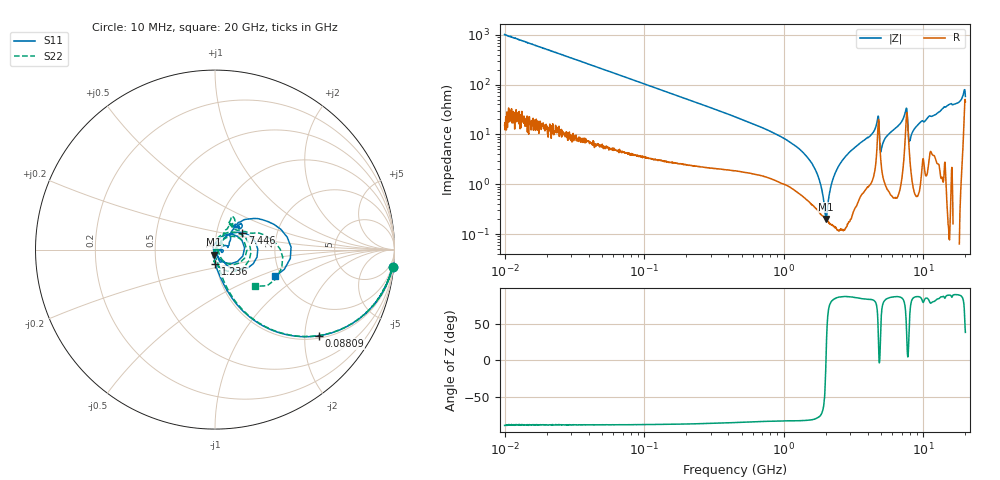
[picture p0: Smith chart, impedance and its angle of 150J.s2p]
!Keysight Technologies,P5008B,MY61100088,A.16.20.02
!Date: Monday, November 06, 2023 16:28:41
!Correction: S11(C  2-Port  )
!S21(C  2-Port  )
!S12(C  2-Port  )
!S22(C  2-Port  )
!S2P File: Measurements: S11, S21, S12, S22:Log Frequency Sweep
# Hz S  dB  R 50
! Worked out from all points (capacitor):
!   1601 points, 10 MHz to 20 GHz, reference 50 ohm
!   read as one part in series: C = 15.7 pF near 10.39 MHz
!   lowest |Z| = 202 mohm at 2.007 GHz (marker M1)
!   series resonance near 2.005 GHz, so ESL is about 400 pH
!   S11 on the Smith chart (normalised r, x): 10 MHz: 1, -20; 88.09 MHz: 1.07, -2.35; 1.236 GHz: 0.99, -0.15; 7.446 GHz: 1.33, +0.26; 20 GHz: 1.87, -0.64
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1e7  -0.05 -5.6  -20.19 83.5  -20.19 83.5  -0.05 -5.6
3.555162e7  -0.56 -18.9  -9.83 69.5  -9.83 69.6  -0.56 -18.9
8.808863e7  -2.48 -39.7  -3.92 48.5  -3.92 48.5  -2.50 -39.7
1.263918e8  -4.07 -49.5  -2.40 38.4  -2.40 38.4  -4.12 -49.5
4.472136e8  -12.78 -73.9  -0.39 12.2  -0.39 12.2  -13.37 -72.9
1.236026e9  -22.21 -89.2  -0.12 2.4  -0.12 2.4  -24.38 -80.4
1.589917e9  -26.09 -94.0  -0.08 0.5  -0.09 0.5  -28.50 -86.5
2.006635e9  -31.16 -98.1  -0.06 -1.4  -0.06 -1.4  -33.15 -97.4
2.681144e9  -41.79 -153.6  -0.07 -4.1  -0.07 -4.1  -41.07 -121.7
3.181218e9  -34.41 121.2  -0.10 -5.7  -0.10 -5.7  -62.47 -44.1
3.565405e9  -30.42 95.1  -0.11 -6.8  -0.11 -6.8  -40.52 54.9
4.696466e9  -17.74 40.3  -0.81 -14.1  -0.81 -14.1  -17.30 31.9
4.901618e9  -23.05 -59.8  -0.41 -5.3  -0.42 -5.3  -21.92 -53.6
5.339198e9  -48.22 -30.4  -0.07 -9.6  -0.08 -9.6  -34.64 4.5
5.652411e9  -40.39 53.8  -0.05 -11.0  -0.06 -11.0  -33.51 44.7
7.445538e9  -14.90 31.8  -0.97 -22.0  -0.98 -22.0  -16.06 36.0
8.626876e9  -31.23 -60.7  -0.05 -16.3  -0.05 -16.3  -32.34 -114.7
9.352484e9  -32.88 -10.2  -0.04 -19.4  -0.04 -19.4  -52.93 174.2
1.099193e10  -24.00 21.4  -0.26 -24.5  -0.26 -24.5  -26.04 34.9
1.374174e10  -16.19 48.2  -0.16 -30.0  -0.16 -30.0  -16.83 59.7
1.871311e10  -13.06 46.6  -0.45 -50.2  -0.45 -50.2  -13.82 28.4
2e10  -8.69 -23.7  -3.64 -39.8  -3.65 -39.8  -10.37 -42.5
